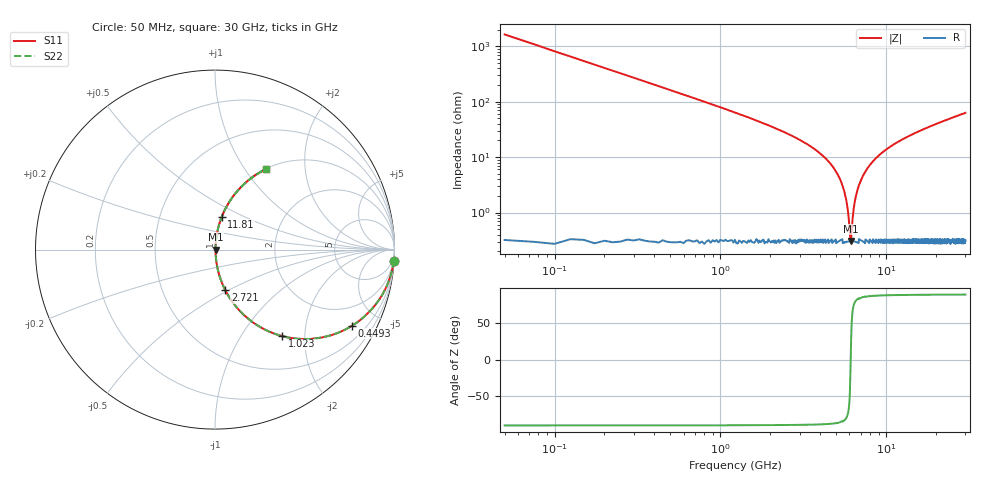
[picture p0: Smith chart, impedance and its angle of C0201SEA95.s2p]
!	AVX Thin Film Operation 	Date: April 2014
!	Description: Accu-P® Series, Thin Film  SMD RF Capacitor
!	Part Number: 02013JA95PBSTR
# MHZ S MA R 50
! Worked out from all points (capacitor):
!   1201 points, 50 MHz to 30 GHz, reference 50 ohm
!   read as one part in series: C = 1.95 pF near 199.8 MHz
!   lowest |Z| = 308 mohm at 6.115 GHz (marker M1)
!   series resonance near 6.103 GHz, so ESL is about 350 pH
!   S11 on the Smith chart (normalised r, x): 50 MHz: 1, -33; 449.3 MHz: 1.01, -3.61; 1.023 GHz: 1.01, -1.55; 2.721 GHz: 1.01, -0.48; 11.81 GHz: 1.01, +0.38; 30 GHz: 1.01, +1.26
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50  0.998 -3.5  0.061 86.5  0.061 86.5  0.998 -3.5
274.625  0.947 -18.6  0.319 71.3  0.319 71.3  0.947 -18.6
449.333  0.874 -28.9  0.484 61.0  0.484 61.0  0.874 -28.9
1023.375  0.611 -52.1  0.789 37.7  0.789 37.7  0.611 -52.1
1697.25  0.405 -65.7  0.912 23.9  0.912 23.9  0.405 -65.7
2720.542  0.233 -75.8  0.97 13.5  0.97 13.5  0.233 -75.8
4118.208  0.107 -82.2  0.991 6.1  0.991 6.1  0.107 -82.2
5041.667  0.051 -83.7  0.996 2.9  0.996 2.9  0.051 -83.7
5590.75  0.024 -81.3  0.997 1.3  0.997 1.3  0.024 -81.3
5790.417  0.014 -77.0  0.997 0.8  0.997 0.8  0.014 -77.0
6015.042  0.004912 -51.5  0.997 0.2  0.997 0.2  0.004912 -51.5
6114.875  0.003087 9.9  0.997 -0.0  0.997 -0.0  0.003087 9.9
6189.75  0.00485 51.0  0.997 -0.2  0.997 -0.2  0.00485 51.0
6564.125  0.02 80.0  0.997 -1.1  0.997 -1.1  0.02 80.0
7188.083  0.044 83.5  0.996 -2.5  0.996 -2.5  0.044 83.5
8286.25  0.083 83.2  0.994 -4.7  0.994 -4.7  0.083 83.2
10058.29  0.138 80.8  0.987 -7.9  0.987 -7.9  0.138 80.8
11805.38  0.186 78.4  0.98 -10.7  0.98 -10.7  0.186 78.4
15025  0.264 74.0  0.961 -15.3  0.961 -15.3  0.264 74.0
20016.67  0.369 67.9  0.927 -21.6  0.927 -21.6  0.369 67.9
25033.29  0.457 62.4  0.887 -27.2  0.887 -27.2  0.457 62.4
30000  0.532 57.6  0.844 -32.1  0.844 -32.1  0.532 57.6
